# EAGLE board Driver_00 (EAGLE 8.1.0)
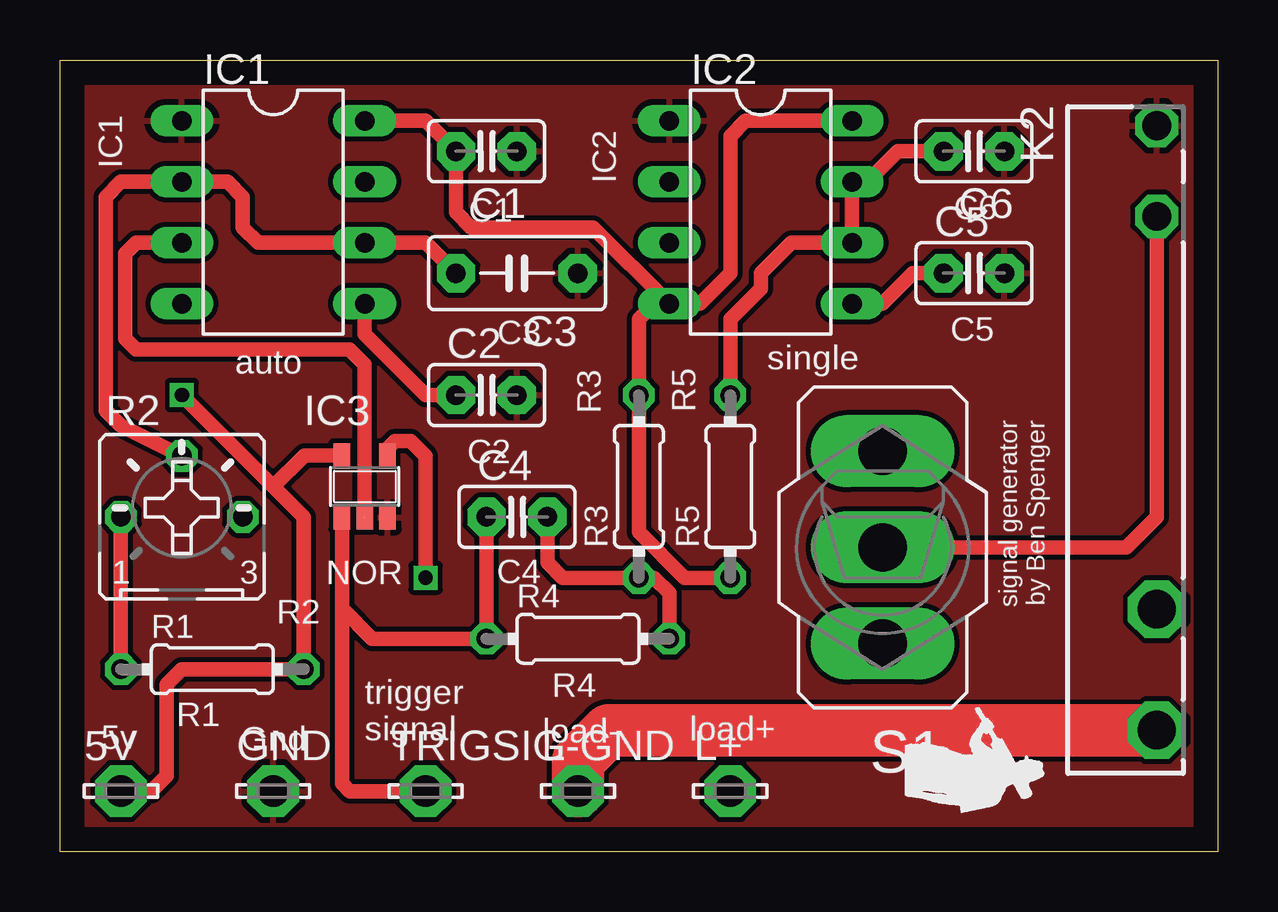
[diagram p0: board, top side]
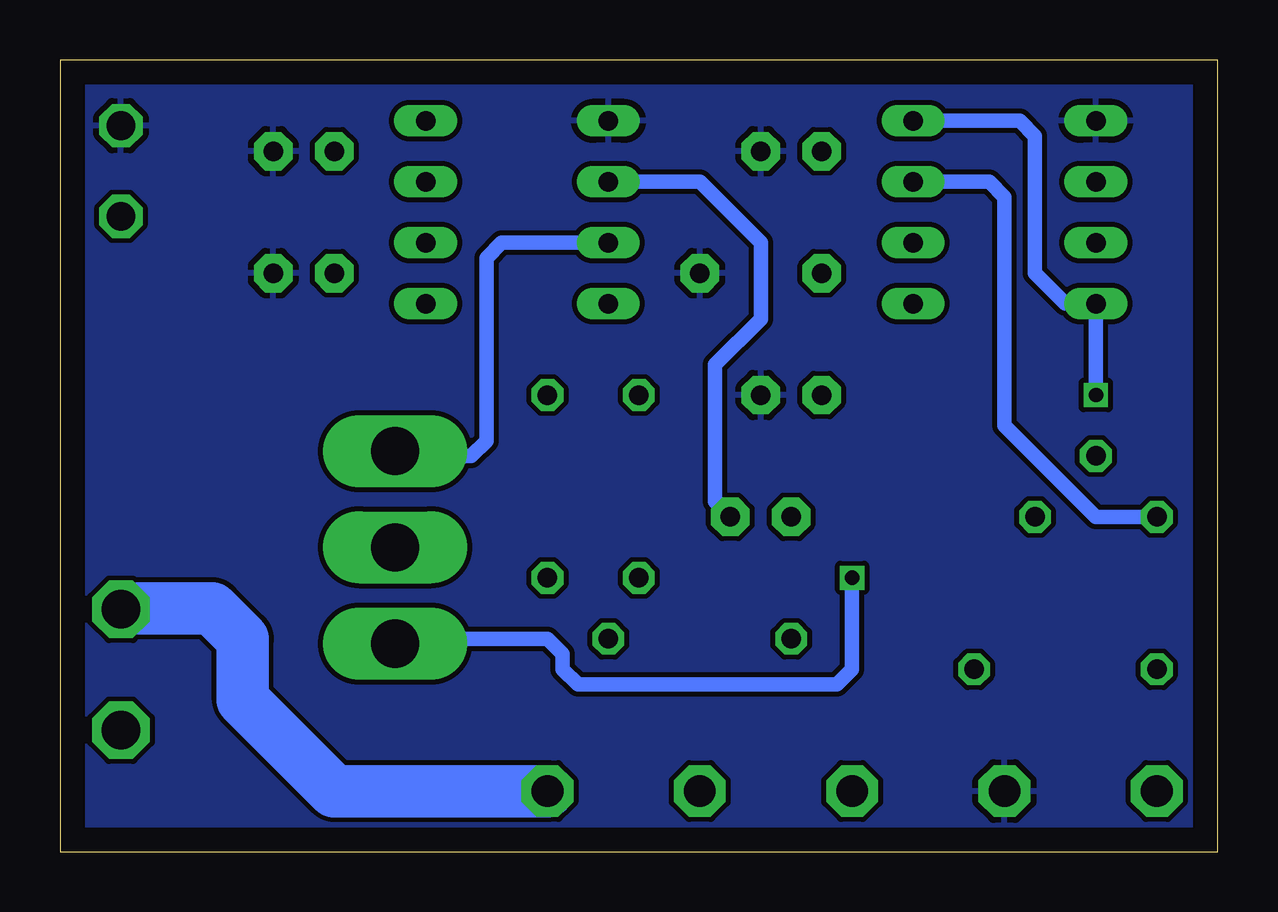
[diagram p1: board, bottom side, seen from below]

Size 48.26 x 33.02 mm. Coordinates in mm from the lower left corner, seen from the top.
Outline: 0,0 0,33.02 48.26,33.02 48.26,0 0,0
Copper layers (1*16): Top 0.035mm / dielectric 1.5mm / Bottom 0.035mm
Design rules "default": minimum track width 10mil, minimum drill 24mil, track to track 8mil, track to pad 8mil, pad to pad 8mil, via to via 8mil, smd to smd 8mil, copper to edge 40mil, drill to drill 8mil, minimum pad ring 10mil, minimum via ring 8mil, stop-mask expansion 4mil, vias tented up to drill 0mil, thermal gap 10mil

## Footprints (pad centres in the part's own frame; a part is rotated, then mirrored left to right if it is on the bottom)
LSP13 = drill 1.321 pad 2.159 octagon: MP 0,0
C2.5-2 = drill 0.813 pad 1.6 octagon: 1 -1.27,0; 2 1.27,0
C5B3 = drill 0.813 pad 1.6 octagon: 1 -2.54,0; 2 2.54,0
DIL-08 = drill 0.813 long: 1 -3.81,-3.81; 2 -1.27,-3.81; 3 1.27,-3.81; 4 3.81,-3.81; 5 3.81,3.81; 6 1.27,3.81; 7 -1.27,3.81; 8 -3.81,3.81
SOT23-5 = smd 0.69 x 0.99: 1 -0.95,-1.29; 2 0,-1.29; 3 0.95,-1.29; 4 0.95,1.3; 5 -0.95,1.3
AQE = drill 1.6 octagon: 3+ 7.66,1.27; 4- 12.7,1.27 | drill 1.2 octagon: I+ -8.72,1.27; I- -12.5,1.27
0204/7 = drill 0.813 octagon: 1 -3.81,0; 2 3.81,0
B25P = drill 0.813 octagon: A -2.54,0; E 2.54,0; S 0,2.54
320-916 = drill 2.007 long: 1 0,4.013; 2 0,0; 3 0,-4.013

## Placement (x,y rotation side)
5V  LSP13  [LSP13]  2.54,2.54 0 top
C1  10nF  [C2.5-2]  17.78,29.21 180 top
C2  0.1uF  [C2.5-2]  17.78,19.05 0 top
C3  470nF  [C5B3]  19.05,24.13 180 top
C4  1uF  [C2.5-2]  19.05,13.97 0 top
C5  0.1uF  [C2.5-2]  38.1,24.13 0 top
C6  0.1uF  [C2.5-2]  38.1,29.21 180 top
GND  LSP13  [LSP13]  8.89,2.54 0 top
IC1  NE555  [DIL-08]  8.89,26.67 270 top
IC2  NE555  [DIL-08]  29.21,26.67 270 top
IC3  NOR  [SOT23-5]  12.7,15.24 0 top
K2  CN024D05  [AQE]  44.45,17.78 270 top
L+  LSP13  [LSP13]  27.94,2.54 0 top
L-GND  LSP13  [LSP13]  21.59,2.54 0 top
R1  390KOhm  [0204/7]  6.35,7.62 0 top
R2  0-1MOhm  [B25P]  5.08,13.97 0 top
R3  10kOhm  [0204/7]  24.13,15.24 90 top
R4  10kOhm  [0204/7]  21.59,8.89 0 top
R5  390 kOhm  [0204/7]  27.94,15.24 90 top
S1  [320-916]  34.29,12.7 180 top
TRIGSIG  LSP13  [LSP13]  15.24,2.54 0 top

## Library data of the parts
5V GND L+ L-GND TRIGSIG = solpad
C1-C6 = capacitor-wima
IC1 IC2 = st-microelectronics; MF: Arrow Electronics; MPN: NE555N; OC_FARNELL: 1467742; OC_NEWARK: 89K1486
IC3 = 74xx-little-us
K2 = CrydomSSR; OC_FARNELL: unknown; OC_NEWARK: unknown
R1 R3-R5 = eagle-ltspice; SPICEMODEL: NONE; SPICEPREFIX: R
R2 = pot
S1 = switch

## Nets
GND: C1.1 C2.2 C3.1 C5.2 C6.1 GND.MP IC1.1 IC2.1 IC3.3 K2.I-
N$1: K2.I+ S1.2
N$2: IC3.4 S1.1
N$3: C3.2 IC1.2 IC1.6 R2.S
N$4: K2.3+ L+.MP
N$5: C2.1 IC1.5
N$6: K2.4- L-GND.MP
N$7: 5V.MP C1.2 IC1.4 IC1.8 IC2.4 IC2.8 IC3.5 R1.2 R3.2 R5.1
N$8: C5.1 IC2.5
N$9: IC1.7 R1.1 R2.A
N$10: IC2.3 S1.3
N$11: C4.2 IC2.2 R3.1 R4.2
N$12: IC1.3 IC3.2
N$14: C6.2 IC2.6 IC2.7 R5.2
N$15: C4.1 IC3.1 R4.1 TRIGSIG.MP

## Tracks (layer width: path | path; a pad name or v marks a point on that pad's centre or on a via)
GND
  pour Bottom (isolate 0.15): 0,33.02 48.26,33.02 48.26,0 0,0
  pour Top (isolate 0.15): 0,33.02 48.26,33.02 48.26,0 0,0
N$1
  Top 0.61: K2.I+ 45.72,13.97 44.45,12.7 S1.2
N$2  (via drill 0.6)
  Top 0.61: IC3.4 13.65,16.83 13.97,17.15 14.6,17.15 15.24,16.51 v15.24,11.43
  Bottom 0.61: v15.24,11.43 15.24,7.62 15.88,6.98 26.67,6.98 27.3,7.62 27.3,8.26 27.94,8.89 34.09,8.89 S1.1
N$3
  Top 0.61: R2.S 2.54,17.78 1.91,18.41 1.91,27.3 2.54,27.94 IC1.2 6.99,27.94 7.62,27.3 7.62,26.03 8.26,25.4 IC1.6 15.24,25.4 C3.2
N$4
  Bottom 2.184: L+.MP 36.83,2.54 40.64,6.35 40.64,8.89 41.91,10.16 45.68,10.16 K2.3+
N$5
  Top 0.61: IC1.5 12.7,21.59 15.24,19.05 C2.1
N$6
  Top 2.184: L-GND.MP 21.59,3.81 22.86,5.08 K2.4-
N$7  (via drill 0.6)
  Top 0.61: IC2.4 24.77,22.86 24.13,22.23 R3.2 24.13,13.33 26.03,11.43 R5.1 | IC1.8 15.24,30.48 C1.2 16.51,26.67 17.15,26.03 22.23,26.03 IC2.4 | IC2.4 26.67,22.86 27.94,24.13 27.94,29.84 28.57,30.48 IC2.8 | 8.89,15.24 10.16,13.97 R1.2 5.08,7.62 4.45,6.98 4.45,3.18 3.81,2.54 5V.MP | 8.89,15.24 v5.08,19.05 | IC3.5 10.19,16.54 8.89,15.24
  Bottom 0.61: IC1.8 8.26,30.48 7.62,29.84 7.62,24.13 6.35,22.86 IC1.4 v5.08,19.05
N$8
  Top 0.61: C5.1 35.56,24.13 34.29,22.86 IC2.5
N$9
  Top 0.61: R1.1 R2.A
  Bottom 0.61: IC1.7 9.53,27.94 8.89,27.3 8.89,17.78 5.08,13.97 R2.A
N$10
  Bottom 0.61: IC2.3 29.84,25.4 30.48,24.77 30.48,17.15 31.12,16.51 34.09,16.51 S1.3
N$11
  Top 0.61: R4.2 25.4,10.79 24.77,11.43 R3.1 20.95,11.43 20.32,12.06 C4.2
  Bottom 0.61: IC2.2 21.59,27.94 19.05,25.4 19.05,22.23 20.95,20.32 20.95,14.6 C4.2
N$12
  Top 0.61: IC3.2 12.7,20.32 12.06,20.95 3.18,20.95 2.72,21.41 2.72,24.94 3.18,25.4 IC1.3
N$14
  Top 0.61: C6.2 34.92,29.21 33.66,27.94 IC2.7 IC2.6 30.48,25.4 29.21,24.13 29.21,23.49 27.94,22.23 R5.2
N$15
  Top 0.61: 11.75,10.16 IC3.1 | 11.75,10.16 11.75,2.85 12.06,2.54 TRIGSIG.MP | C4.1 R4.1 13.02,8.89 11.75,10.16

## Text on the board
tPlace: IC1 | IC2 | C1 | C6 | C3 | C5 | auto | single | R3 | R5 | signal generator / by Ben Spenger | C2 | NOR | C4 | R2 | R4 | R1 | trigger / signal | load- | load+ | 5v | Gnd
